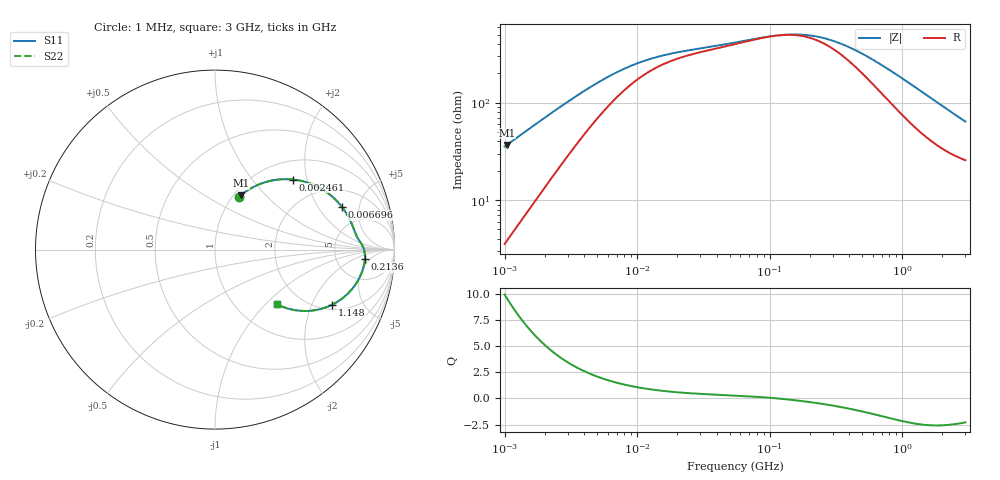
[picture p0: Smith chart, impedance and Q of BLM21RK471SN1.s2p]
! BLM21RK471SN1
# Hz S RI R 50
!Freq.(Hz) S11(Real) S11(Imag) S21(Real) S21(Imag) S12(Real) S12(Imag) S22(Real) S22(Imag)
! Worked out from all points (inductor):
!   401 points, 1 MHz to 3 GHz, reference 50 ohm
!   read as one part in series: L = 5.57 uH near 1.041 MHz
!   highest Q = 9.56 at 1.041 MHz (marker M1), where L = 5.6 uH
!   self-resonance near 115.9 MHz
!   S11 on the Smith chart (normalised r, x): 1 MHz: 1.07, +0.70; 2.461 MHz: 1.40, +1.65; 6.696 MHz: 3.13, +3.35; 213.6 MHz: 10, -4; 1.148 GHz: 2.24, -2.87; 3 GHz: 1.51, -1.17
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1000000  0.1345 0.2945  0.8655 -0.2945  0.8655 -0.2945  0.1345 0.2945
1040844  0.1436 0.3022  0.8564 -0.3022  0.8564 -0.3022  0.1436 0.3022
1682724  0.2887 0.3781  0.7113 -0.3781  0.7113 -0.3781  0.2887 0.3781
2461366  0.4347 0.3905  0.5653 -0.3905  0.5653 -0.3905  0.4347 0.3905
3823119  0.5881 0.3414  0.4119 -0.3414  0.4119 -0.3414  0.5881 0.3414
5059610  0.6589 0.2902  0.3411 -0.2902  0.3411 -0.2902  0.6589 0.2902
6696013  0.7077 0.2371  0.2923 -0.2371  0.2923 -0.2371  0.7077 0.2371
9992459  0.7489 0.1712  0.2511 -0.1712  0.2511 -0.1712  0.7489 0.1712
1.461624e7  0.7696 0.1243  0.2304 -0.1243  0.2304 -0.1243  0.7696 0.1243
2.509235e7  0.7865 0.0809  0.2135 -0.0809  0.2135 -0.0809  0.7865 0.0809
5.477226e7  0.8089 0.0429  0.1911 -0.0429  0.1911 -0.0429  0.8089 0.0429
1.219755e8  0.8315 -0.00374  0.1685 0.00374  0.1685 0.00374  0.8315 -0.00374
1.614254e8  0.8351 -0.0262  0.1649 0.0262  0.1649 0.0262  0.8351 -0.0262
2.094008e8  0.8352 -0.0505  0.1648 0.0505  0.1648 0.0505  0.8352 -0.0505
2.136344e8  0.8351 -0.0525  0.1649 0.0525  0.1649 0.0525  0.8351 -0.0525
2.827291e8  0.8308 -0.0833  0.1692 0.0833  0.1692 0.0833  0.8308 -0.0833
3.741707e8  0.8207 -0.1197  0.1793 0.1197  0.1793 0.1197  0.8207 -0.1197
5.583748e8  0.7906 -0.1824  0.2094 0.1824  0.2094 0.1824  0.7906 -0.1824
8.005644e8  0.7386 -0.2466  0.2614 0.2466  0.2614 0.2466  0.7386 -0.2466
1.147801e9  0.6544 -0.3061  0.3456 0.3061  0.3456 0.3061  0.6544 -0.3061
1.855641e9  0.4991 -0.3421  0.5009 0.3421  0.5009 0.3421  0.4991 -0.3421
3e9  0.3461 -0.3046  0.6539 0.3046  0.6539 0.3046  0.3461 -0.3046
